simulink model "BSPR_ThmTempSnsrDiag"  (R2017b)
settings: Solver=FixedStepDiscrete  StartTime=0.0  StopTime=10.0  FixedStep=0.02  RelTol=1e-3  EnableMultiTasking=on
undefined symbols (not defined in the file): BCCR_cntClntTempDiag_CW, bin2dec, BSPR_tClntDsTOvrTemp_C, BSPR_tClntUsTOvrTemp_C, BSPR_tiClntDsTElecMax_C, BSPR_tiClntDsTElecMin_C, BSPR_tiClntDsTJit_C, BSPR_tiClntDsTOvrTemp_C, BSPR_tiClntDsTVld_C, BSPR_tiClntUsTElecMax_C, BSPR_tiClntUsTElecMin_C, BSPR_tiClntUsTJit_C, BSPR_tiClntUsTOvrTemp_C, BSPR_tiClntUsTVld_C, BSPR_uClntDsTElecMax_C, BSPR_uClntDsTElecMin_C, BSPR_uClntDsTJitDiff_C, BSPR_uClntUsTElecMax_C, BSPR_uClntUsTElecMin_C, BSPR_uClntUsTJitDiff_C
libraries: simulink x64
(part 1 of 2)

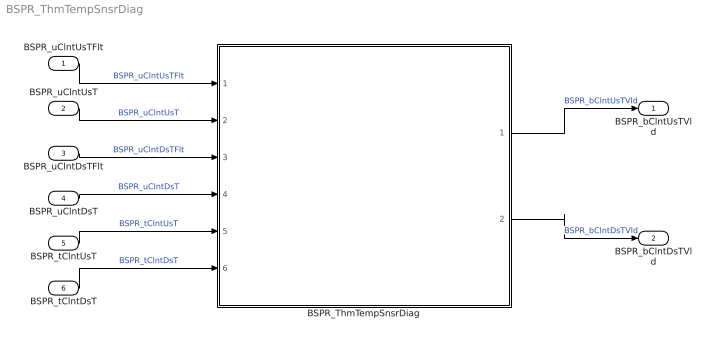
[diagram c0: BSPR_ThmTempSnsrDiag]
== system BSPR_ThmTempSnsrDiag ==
  BSPR_uClntUsTFlt : Inport
  BSPR_uClntUsT : Inport  Port=2
  BSPR_uClntDsTFlt : Inport  Port=3
  BSPR_uClntDsT : Inport  Port=4
  BSPR_tClntUsT : Inport  Port=5
  BSPR_tClntDsT : Inport  Port=6
  BSPR_ThmTempSnsrDiag : Subsystem
  BSPR_bClntUsTVld : Outport
  BSPR_bClntDsTVld : Outport  Port=2
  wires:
  BSPR_uClntUsTFlt/1 -> BSPR_ThmTempSnsrDiag/1(BSPR_uClntUsTFlt)  "BSPR_uClntUsTFlt"
  BSPR_uClntUsT/1 -> BSPR_ThmTempSnsrDiag/2(BSPR_uClntUsT)  "BSPR_uClntUsT"
  BSPR_uClntDsTFlt/1 -> BSPR_ThmTempSnsrDiag/3(BSPR_uClntDsTFlt)  "BSPR_uClntDsTFlt"
  BSPR_uClntDsT/1 -> BSPR_ThmTempSnsrDiag/4(BSPR_uClntDsT)  "BSPR_uClntDsT"
  BSPR_ThmTempSnsrDiag/1(BSPR_bClntUsTVld) -> BSPR_bClntUsTVld/1  "BSPR_bClntUsTVld"
  BSPR_ThmTempSnsrDiag/2(BSPR_bClntDsTVld) -> BSPR_bClntDsTVld/1  "BSPR_bClntDsTVld"
  BSPR_tClntUsT/1 -> BSPR_ThmTempSnsrDiag/5(BSPR_tClntUsT)  "BSPR_tClntUsT"
  BSPR_tClntDsT/1 -> BSPR_ThmTempSnsrDiag/6(BSPR_tClntDsT)  "BSPR_tClntDsT"

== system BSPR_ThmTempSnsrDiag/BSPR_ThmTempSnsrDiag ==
  BSPR_uClntUsTFlt : Inport
  BSPR_uClntUsT : Inport  Port=2
  BSPR_uClntDsTFlt : Inport  Port=3
  BSPR_uClntDsT : Inport  Port=4
  BSPR_tClntUsT : Inport  Port=5
  BSPR_tClntDsT : Inport  Port=6
  CIntDsTErrChk : Subsystem
  CIntTempDsmRpt : Subsystem
  CIntUsTErrChk : Subsystem
  BSPR_bClntUsTVld : Outport
  BSPR_bClntDsTVld : Outport  Port=2
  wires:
  BSPR_uClntUsTFlt/1 -> CIntUsTErrChk/1(BSPR_uClntUsTFlt)
  BSPR_uClntUsT/1 -> CIntUsTErrChk/2(BSPR_uClntUsT)
  CIntUsTErrChk/1(BSPR_bClntUsTJitErrStt) -> CIntTempDsmRpt/1(BSPR_bClntUsTJitErrStt)
  CIntUsTErrChk/2(BSPR_bClntUsTMaxErrStt) -> CIntTempDsmRpt/2(BSPR_bClntUsTMaxErrStt)
  CIntUsTErrChk/3(BSPR_bClntUsTMinErrStt) -> CIntTempDsmRpt/3(BSPR_bClntUsTMinErrStt)
  CIntUsTErrChk/4(BSPR_bClntUsTJitErrDet) -> CIntTempDsmRpt/4(BSPR_bClntUsTJitErrDet)
  CIntUsTErrChk/5(BSPR_bClntUsTJitErrHeal) -> CIntTempDsmRpt/5(BSPR_bClntUsTJitErrHeal)
  CIntUsTErrChk/6(BSPR_bClntUsTMaxErrDet) -> CIntTempDsmRpt/6(BSPR_bClntUsTMaxErrDet)
  CIntUsTErrChk/7(BSPR_bClntUsTMaxErrHeal) -> CIntTempDsmRpt/7(BSPR_bClntUsTMaxErrHeal)
  CIntUsTErrChk/8(BSPR_bClntUsTMinErrDet) -> CIntTempDsmRpt/8(BSPR_bClntUsTMinErrDet)
  CIntUsTErrChk/9(BSPR_bClntUsTMinErrHeal) -> CIntTempDsmRpt/9(BSPR_bClntUsTMinErrHeal)
  CIntTempDsmRpt/1(BSPR_bClntUsTVld) -> BSPR_bClntUsTVld/1
  BSPR_uClntDsTFlt/1 -> CIntDsTErrChk/2(BSPR_uClntDsTFlt)
  BSPR_uClntDsT/1 -> CIntDsTErrChk/3(BSPR_uClntDsT)
  CIntTempDsmRpt/2(BSPR_bClntDsTVld) -> BSPR_bClntDsTVld/1
  CIntDsTErrChk/1(BSPR_bClntDsTJitErrStt) -> CIntTempDsmRpt/12(BSPR_bClntDsTJitErrStt)
  CIntDsTErrChk/2(BSPR_bClntDsTMaxErrStt) -> CIntTempDsmRpt/13(BSPR_bClntDsTMaxErrStt)
  CIntDsTErrChk/3(BSPR_bClntDsTMinErrStt) -> CIntTempDsmRpt/14(BSPR_bClntDsTMinErrStt)
  CIntDsTErrChk/4(BSPR_bClntDsTJitErrDet) -> CIntTempDsmRpt/15(BSPR_bClntDsTJitErrDet)
  CIntDsTErrChk/5(BSPR_bClntDsTJitErrHeal) -> CIntTempDsmRpt/16(BSPR_bClntDsTJitErrHeal)
  CIntDsTErrChk/6(BSPR_bClntDsTMaxErrDet) -> CIntTempDsmRpt/17(BSPR_bClntDsTMaxErrDet)
  CIntDsTErrChk/7(BSPR_bClntDsTMaxErrHeal) -> CIntTempDsmRpt/18(BSPR_bClntDsTMaxErrHeal)
  CIntDsTErrChk/8(BSPR_bClntDsTMinErrDet) -> CIntTempDsmRpt/19(BSPR_bClntDsTMinErrDet)
  CIntDsTErrChk/9(BSPR_bClntDsTMinErrHeal) -> CIntTempDsmRpt/20(BSPR_bClntDsTMinErrHeal)
  BSPR_tClntUsT/1 -> CIntUsTErrChk/3(BSPR_tClntUsT)
  BSPR_tClntDsT/1 -> CIntDsTErrChk/1(BSPR_tClntDsT)
  CIntUsTErrChk/10(BSPR_bClntUsTOTErrDet) -> CIntTempDsmRpt/10(BSPR_bClntUsTOTErrDet)
  CIntUsTErrChk/11(BSPR_bClntUsTOTErrHeal) -> CIntTempDsmRpt/11(BSPR_bClntUsTOTErrHeal)
  CIntDsTErrChk/10(BSPR_bClntDsTOTErrDet) -> CIntTempDsmRpt/21(BSPR_bClntDsTOTErrDet)
  CIntDsTErrChk/11(BSPR_bClntDsTOTErrHeal) -> CIntTempDsmRpt/22(BSPR_bClntDsTOTErrHeal)

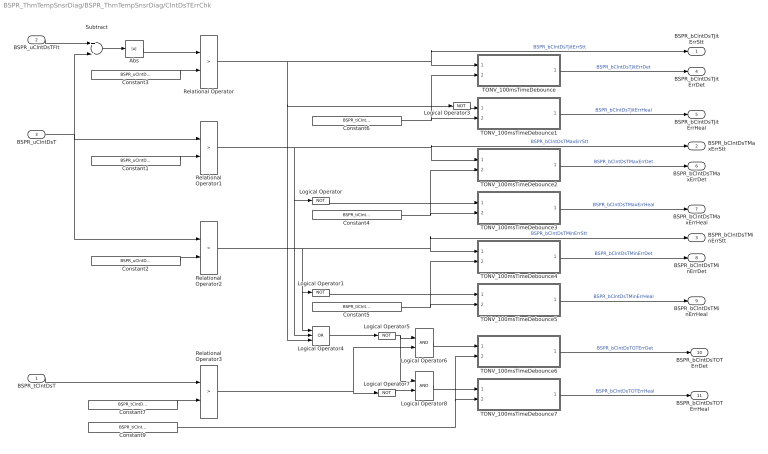
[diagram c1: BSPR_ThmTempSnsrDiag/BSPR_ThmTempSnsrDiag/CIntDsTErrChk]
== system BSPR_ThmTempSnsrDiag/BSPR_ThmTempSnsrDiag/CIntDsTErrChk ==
  BSPR_tClntDsT : Inport
  BSPR_uClntDsTFlt : Inport  Port=2
  BSPR_uClntDsT : Inport  Port=3
  Abs : Abs
  Constant1 : Constant  Value=BSPR_uClntDsTElecMax_C  OutDataTypeStr=single
  Constant2 : Constant  Value=BSPR_uClntDsTElecMin_C  OutDataTypeStr=single
  Constant3 : Constant  Value=BSPR_uClntDsTJitDiff_C  OutDataTypeStr=single
  Constant4 : Constant  Value=BSPR_tiClntDsTElecMax_C  OutDataTypeStr=single
  Constant5 : Constant  Value=BSPR_tiClntDsTElecMin_C  OutDataTypeStr=single
  Constant6 : Constant  Value=BSPR_tiClntDsTJit_C  OutDataTypeStr=single
  Constant7 : Constant  Value=BSPR_tClntDsTOvrTemp_C  OutDataTypeStr=single
  Constant9 : Constant  Value=BSPR_tiClntDsTOvrTemp_C  OutDataTypeStr=single
  Logical Operator{,1,3,5,7} (5 alike) : Logic  Operator=NOT  AllPortsSameDT=off  OutDataTypeStr=boolean
  Logical Operator4 : Logic  Operator=OR  Inputs=3  AllPortsSameDT=off  OutDataTypeStr=boolean
  Logical Operator6 : Logic  AllPortsSameDT=off  OutDataTypeStr=boolean
  Logical Operator8 : Logic  AllPortsSameDT=off  OutDataTypeStr=boolean
  Relational Operator : RelationalOperator  Operator=>  OutDataTypeStr=boolean  RndMeth=Simplest
  Relational Operator1 : RelationalOperator  Operator=>  OutDataTypeStr=boolean  RndMeth=Simplest
  Relational Operator2 : RelationalOperator  Operator=<  OutDataTypeStr=boolean  RndMeth=Simplest
  Relational Operator3 : RelationalOperator  Operator=>  OutDataTypeStr=boolean  RndMeth=Simplest
  Subtract : Sum  Inputs=+-
  TONV_100msTimeDebounce : Subsystem  TreatAsAtomicUnit=on  RTWFcnName=TONV_100msTimeDebounce  RTWFileName=SrvLib
  TONV_100msTimeDebounce1 : Subsystem  TreatAsAtomicUnit=on  RTWFcnName=TONV_100msTimeDebounce  RTWFileName=SrvLib
  TONV_100msTimeDebounce2 : Subsystem  TreatAsAtomicUnit=on  RTWFcnName=TONV_100msTimeDebounce  RTWFileName=SrvLib
  TONV_100msTimeDebounce3 : Subsystem  TreatAsAtomicUnit=on  RTWFcnName=TONV_100msTimeDebounce  RTWFileName=SrvLib
  TONV_100msTimeDebounce4 : Subsystem  TreatAsAtomicUnit=on  RTWFcnName=TONV_100msTimeDebounce  RTWFileName=SrvLib
  TONV_100msTimeDebounce5 : Subsystem  TreatAsAtomicUnit=on  RTWFcnName=TONV_100msTimeDebounce  RTWFileName=SrvLib
  TONV_100msTimeDebounce6 : Subsystem  TreatAsAtomicUnit=on  RTWFcnName=TONV_100msTimeDebounce  RTWFileName=SrvLib
  TONV_100msTimeDebounce7 : Subsystem  TreatAsAtomicUnit=on  RTWFcnName=TONV_100msTimeDebounce  RTWFileName=SrvLib
  BSPR_bClntDsTJitErrStt : Outport
  BSPR_bClntDsTMaxErrStt : Outport  Port=2
  BSPR_bClntDsTMinErrStt : Outport  Port=3
  BSPR_bClntDsTJitErrDet : Outport  Port=4
  BSPR_bClntDsTJitErrHeal : Outport  Port=5
  BSPR_bClntDsTMaxErrDet : Outport  Port=6
  BSPR_bClntDsTMaxErrHeal : Outport  Port=7
  BSPR_bClntDsTMinErrDet : Outport  Port=8
  BSPR_bClntDsTMinErrHeal : Outport  Port=9
  BSPR_bClntDsTOTErrDet : Outport  Port=10
  BSPR_bClntDsTOTErrHeal : Outport  Port=11
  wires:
  TONV_100msTimeDebounce2/1(y) -> BSPR_bClntDsTMaxErrDet/1  "BSPR_bClntDsTMaxErrDet"
  TONV_100msTimeDebounce1/1(y) -> BSPR_bClntDsTJitErrHeal/1  "BSPR_bClntDsTJitErrHeal"
  TONV_100msTimeDebounce3/1(y) -> BSPR_bClntDsTMaxErrHeal/1  "BSPR_bClntDsTMaxErrHeal"
  TONV_100msTimeDebounce4/1(y) -> BSPR_bClntDsTMinErrDet/1  "BSPR_bClntDsTMinErrDet"
  Logical Operator/1 -> TONV_100msTimeDebounce3/1(u)
  Constant4/1 -> TONV_100msTimeDebounce2/2(T), TONV_100msTimeDebounce3/2(T)
  BSPR_uClntDsT/1 -> Relational Operator2/1, Relational Operator1/1, Subtract/2
  Relational Operator1/1 -> TONV_100msTimeDebounce2/1(u), BSPR_bClntDsTMaxErrStt/1, Logical Operator4/2, Logical Operator/1  "BSPR_bClntDsTMaxErrStt"
  Constant1/1 -> Relational Operator1/2
  Constant2/1 -> Relational Operator2/2
  Constant6/1 -> TONV_100msTimeDebounce/2(T), TONV_100msTimeDebounce1/2(T)
  Relational Operator/1 -> TONV_100msTimeDebounce/1(u), BSPR_bClntDsTJitErrStt/1, Logical Operator4/3, Logical Operator3/1  "BSPR_bClntDsTJitErrStt"
  BSPR_uClntDsTFlt/1 -> Subtract/1
  Subtract/1 -> Abs/1
  Abs/1 -> Relational Operator/1
  Constant3/1 -> Relational Operator/2
  TONV_100msTimeDebounce/1(y) -> BSPR_bClntDsTJitErrDet/1  "BSPR_bClntDsTJitErrDet"
  Constant5/1 -> TONV_100msTimeDebounce4/2(T), TONV_100msTimeDebounce5/2(T)
  TONV_100msTimeDebounce5/1(y) -> BSPR_bClntDsTMinErrHeal/1  "BSPR_bClntDsTMinErrHeal"
  Logical Operator1/1 -> TONV_100msTimeDebounce5/1(u)
  Relational Operator2/1 -> Logical Operator4/1, Logical Operator1/1, BSPR_bClntDsTMinErrStt/1, TONV_100msTimeDebounce4/1(u)  "BSPR_bClntDsTMinErrStt"
  Logical Operator3/1 -> TONV_100msTimeDebounce1/1(u)
  Logical Operator4/1 -> Logical Operator5/1
  Constant7/1 -> Relational Operator3/2
  BSPR_tClntDsT/1 -> Relational Operator3/1
  Logical Operator5/1 -> Logical Operator8/1, Logical Operator6/1
  Relational Operator3/1 -> Logical Operator6/2, Logical Operator7/1
  Logical Operator6/1 -> TONV_100msTimeDebounce6/1(u)
  Logical Operator8/1 -> TONV_100msTimeDebounce7/1(u)
  Constant9/1 -> TONV_100msTimeDebounce6/2(T), TONV_100msTimeDebounce7/2(T)
  TONV_100msTimeDebounce6/1(y) -> BSPR_bClntDsTOTErrDet/1  "BSPR_bClntDsTOTErrDet"
  TONV_100msTimeDebounce7/1(y) -> BSPR_bClntDsTOTErrHeal/1  "BSPR_bClntDsTOTErrHeal"
  Logical Operator7/1 -> Logical Operator8/2

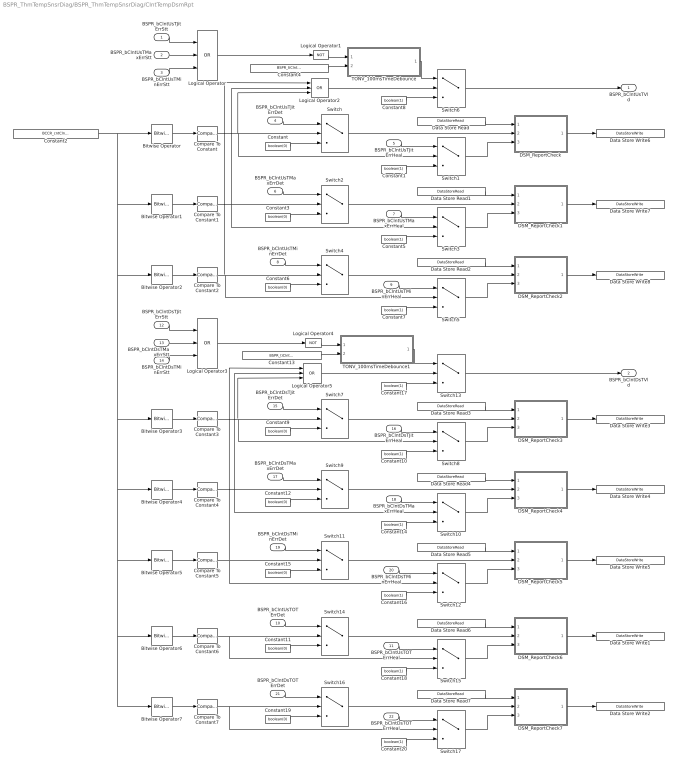
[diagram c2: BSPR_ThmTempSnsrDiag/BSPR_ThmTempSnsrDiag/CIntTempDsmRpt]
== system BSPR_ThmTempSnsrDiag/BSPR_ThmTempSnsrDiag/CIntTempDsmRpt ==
  BSPR_bClntUsTJitErrStt : Inport
  BSPR_bClntUsTMaxErrStt : Inport  Port=2
  BSPR_bClntUsTMinErrStt : Inport  Port=3
  BSPR_bClntUsTJitErrDet : Inport  Port=4
  BSPR_bClntUsTJitErrHeal : Inport  Port=5
  BSPR_bClntUsTMaxErrDet : Inport  Port=6
  BSPR_bClntUsTMaxErrHeal : Inport  Port=7
  BSPR_bClntUsTMinErrDet : Inport  Port=8
  BSPR_bClntUsTMinErrHeal : Inport  Port=9
  BSPR_bClntUsTOTErrDet : Inport  Port=10
  BSPR_bClntUsTOTErrHeal : Inport  Port=11
  BSPR_bClntDsTJitErrStt : Inport  Port=12
  BSPR_bClntDsTMaxErrStt : Inport  Port=13
  BSPR_bClntDsTMinErrStt : Inport  Port=14
  BSPR_bClntDsTJitErrDet : Inport  Port=15
  BSPR_bClntDsTJitErrHeal : Inport  Port=16
  BSPR_bClntDsTMaxErrDet : Inport  Port=17
  BSPR_bClntDsTMaxErrHeal : Inport  Port=18
  BSPR_bClntDsTMinErrDet : Inport  Port=19
  BSPR_bClntDsTMinErrHeal : Inport  Port=20
  BSPR_bClntDsTOTErrDet : Inport  Port=21
  BSPR_bClntDsTOTErrHeal : Inport  Port=22
  Bitwise Operator : simulink/Logic and Bit Operations/Bitwise Operator  logicop=AND  UseBitMask=on  BitMask=bin2dec('00000001')  BitMaskRealWorld=Stored Integer
  Bitwise Operator1 : simulink/Logic and Bit Operations/Bitwise Operator  logicop=AND  UseBitMask=on  BitMask=bin2dec('00000010')  BitMaskRealWorld=Stored Integer
  Bitwise Operator2 : simulink/Logic and Bit Operations/Bitwise Operator  logicop=AND  UseBitMask=on  BitMask=bin2dec('00000100')  BitMaskRealWorld=Stored Integer
  Bitwise Operator3 : simulink/Logic and Bit Operations/Bitwise Operator  logicop=AND  UseBitMask=on  BitMask=bin2dec('00001000')  BitMaskRealWorld=Stored Integer
  Bitwise Operator4 : simulink/Logic and Bit Operations/Bitwise Operator  logicop=AND  UseBitMask=on  BitMask=bin2dec('00010000')  BitMaskRealWorld=Stored Integer
  Bitwise Operator5 : simulink/Logic and Bit Operations/Bitwise Operator  logicop=AND  UseBitMask=on  BitMask=bin2dec('00100000')  BitMaskRealWorld=Stored Integer
  Bitwise Operator6 : simulink/Logic and Bit Operations/Bitwise Operator  logicop=AND  UseBitMask=on  BitMask=bin2dec('01000000')  BitMaskRealWorld=Stored Integer
  Bitwise Operator7 : simulink/Logic and Bit Operations/Bitwise Operator  logicop=AND  UseBitMask=on  BitMask=bin2dec('10000000')  BitMaskRealWorld=Stored Integer
  Compare To Constant : simulink/Logic and Bit Operations/Compare To Constant  relop===  const=1  OutDataTypeStr=boolean
  Compare To Constant1 : simulink/Logic and Bit Operations/Compare To Constant  relop===  const=2  OutDataTypeStr=boolean
  Compare To Constant2 : simulink/Logic and Bit Operations/Compare To Constant  relop===  const=4  OutDataTypeStr=boolean
  Compare To Constant3 : simulink/Logic and Bit Operations/Compare To Constant  relop===  const=8  OutDataTypeStr=boolean
  Compare To Constant4 : simulink/Logic and Bit Operations/Compare To Constant  relop===  const=16  OutDataTypeStr=boolean
  Compare To Constant5 : simulink/Logic and Bit Operations/Compare To Constant  relop===  const=32  OutDataTypeStr=boolean
  Compare To Constant6 : simulink/Logic and Bit Operations/Compare To Constant  relop===  const=64  OutDataTypeStr=boolean
  Compare To Constant7 : simulink/Logic and Bit Operations/Compare To Constant  relop===  const=128  OutDataTypeStr=boolean
  Constant{,3,6,9,11..12,15,19} (8 alike) : Constant  Value=boolean(0)  OutDataTypeStr=boolean
  Constant{1,5,7..8,10,14,16..18,20} (10 alike) : Constant  Value=boolean(1)  OutDataTypeStr=boolean
  Constant13 : Constant  Value=BSPR_tiClntDsTVld_C  OutDataTypeStr=single
  Constant2 : Constant  Value=BCCR_cntClntTempDiag_CW
  Constant4 : Constant  Value=BSPR_tiClntUsTVld_C  OutDataTypeStr=single
  DSM_ReportCheck : Subsystem  TreatAsAtomicUnit=on  RTWFcnName=DSM_ReportCheck  RTWFileName=SrvLib
  DSM_ReportCheck1 : Subsystem  TreatAsAtomicUnit=on  RTWFcnName=DSM_ReportCheck  RTWFileName=SrvLib
  DSM_ReportCheck2 : Subsystem  TreatAsAtomicUnit=on  RTWFcnName=DSM_ReportCheck  RTWFileName=SrvLib
  DSM_ReportCheck3 : Subsystem  TreatAsAtomicUnit=on  RTWFcnName=DSM_ReportCheck  RTWFileName=SrvLib
  DSM_ReportCheck4 : Subsystem  TreatAsAtomicUnit=on  RTWFcnName=DSM_ReportCheck  RTWFileName=SrvLib
  DSM_ReportCheck5 : Subsystem  TreatAsAtomicUnit=on  RTWFcnName=DSM_ReportCheck  RTWFileName=SrvLib
  DSM_ReportCheck6 : Subsystem  TreatAsAtomicUnit=on  RTWFcnName=DSM_ReportCheck  RTWFileName=SrvLib
  DSM_ReportCheck7 : Subsystem  TreatAsAtomicUnit=on  RTWFcnName=DSM_ReportCheck  RTWFileName=SrvLib
  Data Store Read : DataStoreRead  DataStoreName=DFC_ClntUsTElecSig
  Data Store Read1 : DataStoreRead  DataStoreName=DFC_ClntUsTElecMax
  Data Store Read2 : DataStoreRead  DataStoreName=DFC_ClntUsTElecMin
  Data Store Read3 : DataStoreRead  DataStoreName=DFC_ClntDsTElecSig
  Data Store Read4 : DataStoreRead  DataStoreName=DFC_ClntDsTElecMax
  Data Store Read5 : DataStoreRead  DataStoreName=DFC_ClntDsTElecMin
  Data Store Read6 : DataStoreRead  DataStoreName=DFC_InClntOverTmp
  Data Store Read7 : DataStoreRead  DataStoreName=DFC_OutClntOverTmp
  Data Store Write1 : DataStoreWrite  DataStoreName=DFC_InClntOverTmp
  Data Store Write2 : DataStoreWrite  DataStoreName=DFC_OutClntOverTmp
  Data Store Write3 : DataStoreWrite  DataStoreName=DFC_ClntDsTElecSig
  Data Store Write4 : DataStoreWrite  DataStoreName=DFC_ClntDsTElecMax
  Data Store Write5 : DataStoreWrite  DataStoreName=DFC_ClntDsTElecMin
  Data Store Write6 : DataStoreWrite  DataStoreName=DFC_ClntUsTElecSig
  Data Store Write7 : DataStoreWrite  DataStoreName=DFC_ClntUsTElecMax
  Data Store Write8 : DataStoreWrite  DataStoreName=DFC_ClntUsTElecMin
  Logical Operator{,2..3,5} (4 alike) : Logic  Operator=OR  Inputs=3  AllPortsSameDT=off  OutDataTypeStr=boolean
  Logical Operator1 : Logic  Operator=NOT  AllPortsSameDT=off  OutDataTypeStr=boolean
  Logical Operator4 : Logic  Operator=NOT  AllPortsSameDT=off  OutDataTypeStr=boolean
  Switch{,1..17} (18 alike) : Switch  Criteria=u2 > Threshold
  TONV_100msTimeDebounce : Subsystem  TreatAsAtomicUnit=on  RTWFcnName=TONV_100msTimeDebounce  RTWFileName=SrvLib
  TONV_100msTimeDebounce1 : Subsystem  TreatAsAtomicUnit=on  RTWFcnName=TONV_100msTimeDebounce  RTWFileName=SrvLib
  BSPR_bClntUsTVld : Outport
  BSPR_bClntDsTVld : Outport  Port=2
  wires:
  BSPR_bClntUsTJitErrStt/1 -> Logical Operator/1
  BSPR_bClntUsTMaxErrStt/1 -> Logical Operator/2
  BSPR_bClntUsTMinErrStt/1 -> Logical Operator/3
  Logical Operator/1 -> Logical Operator1/1
  Logical Operator1/1 -> TONV_100msTimeDebounce/1(u)
  Switch6/1 -> BSPR_bClntUsTVld/1
  Constant4/1 -> TONV_100msTimeDebounce/2(T)
  Constant/1 -> Switch/3
  BSPR_bClntUsTJitErrDet/1 -> Switch/1
  BSPR_bClntUsTJitErrHeal/1 -> Switch1/1
  Constant1/1 -> Switch1/3
  Switch1/1 -> DSM_ReportCheck/3(Heal)
  Switch/1 -> DSM_ReportCheck/2(Err)
  Bitwise Operator/1 -> Compare To Constant/1
  Compare To Constant/1 -> Logical Operator2/3, Switch1/2, Switch/2
  Constant3/1 -> Switch2/3
  Constant5/1 -> Switch3/3
  Switch3/1 -> DSM_ReportCheck1/3(Heal)
  Switch2/1 -> DSM_ReportCheck1/2(Err)
  BSPR_bClntUsTMaxErrHeal/1 -> Switch3/1
  BSPR_bClntUsTMaxErrDet/1 -> Switch2/1
  Bitwise Operator1/1 -> Compare To Constant1/1
  Compare To Constant1/1 -> Switch2/2, Switch3/2, Logical Operator2/2
  Data Store Read1/1 -> DSM_ReportCheck1/1(Dfc_id_nv)
  Data Store Read/1 -> DSM_ReportCheck/1(Dfc_id_nv)
  Constant6/1 -> Switch4/3
  Constant7/1 -> Switch5/3
  Switch5/1 -> DSM_ReportCheck2/3(Heal)
  Switch4/1 -> DSM_ReportCheck2/2(Err)
  BSPR_bClntUsTMinErrHeal/1 -> Switch5/1
  BSPR_bClntUsTMinErrDet/1 -> Switch4/1
  Bitwise Operator2/1 -> Compare To Constant2/1
  Compare To Constant2/1 -> Switch4/2, Switch5/2, Logical Operator2/1
  Data Store Read2/1 -> DSM_ReportCheck2/1(Dfc_id_nv)
  DSM_ReportCheck/1(Dfc_id) -> Data Store Write6/1
  DSM_ReportCheck1/1(Dfc_id) -> Data Store Write7/1
  DSM_ReportCheck2/1(Dfc_id) -> Data Store Write8/1
  TONV_100msTimeDebounce/1(y) -> Switch6/1
  Constant8/1 -> Switch6/3
  Logical Operator2/1 -> Switch6/2
  Logical Operator5/1 -> Switch13/2
  Constant17/1 -> Switch13/3
  TONV_100msTimeDebounce1/1(y) -> Switch13/1
  DSM_ReportCheck5/1(Dfc_id) -> Data Store Write5/1
  DSM_ReportCheck4/1(Dfc_id) -> Data Store Write4/1
  DSM_ReportCheck3/1(Dfc_id) -> Data Store Write3/1
  Data Store Read5/1 -> DSM_ReportCheck5/1(Dfc_id_nv)
  Compare To Constant5/1 -> Switch11/2, Switch12/2, Logical Operator5/1
  Bitwise Operator5/1 -> Compare To Constant5/1
  BSPR_bClntDsTMinErrDet/1 -> Switch11/1
  BSPR_bClntDsTMinErrHeal/1 -> Switch12/1
  Switch11/1 -> DSM_ReportCheck5/2(Err)
  Switch12/1 -> DSM_ReportCheck5/3(Heal)
  Constant16/1 -> Switch12/3
  Constant15/1 -> Switch11/3
  Data Store Read3/1 -> DSM_ReportCheck3/1(Dfc_id_nv)
  Data Store Read4/1 -> DSM_ReportCheck4/1(Dfc_id_nv)
  Compare To Constant4/1 -> Switch9/2, Switch10/2, Logical Operator5/2
  Bitwise Operator4/1 -> Compare To Constant4/1
  BSPR_bClntDsTMaxErrDet/1 -> Switch9/1
  BSPR_bClntDsTMaxErrHeal/1 -> Switch10/1
  Switch9/1 -> DSM_ReportCheck4/2(Err)
  Switch10/1 -> DSM_ReportCheck4/3(Heal)
  Constant14/1 -> Switch10/3
  Constant12/1 -> Switch9/3
  Compare To Constant3/1 -> Logical Operator5/3, Switch7/2, Switch8/2
  Bitwise Operator3/1 -> Compare To Constant3/1
  Switch7/1 -> DSM_ReportCheck3/2(Err)
  Switch8/1 -> DSM_ReportCheck3/3(Heal)
  Constant10/1 -> Switch8/3
  BSPR_bClntDsTJitErrHeal/1 -> Switch8/1
  BSPR_bClntDsTJitErrDet/1 -> Switch7/1
  Constant9/1 -> Switch7/3
  Constant13/1 -> TONV_100msTimeDebounce1/2(T)
  Switch13/1 -> BSPR_bClntDsTVld/1
  Logical Operator4/1 -> TONV_100msTimeDebounce1/1(u)
  Logical Operator3/1 -> Logical Operator4/1
  BSPR_bClntDsTMinErrStt/1 -> Logical Operator3/3
  BSPR_bClntDsTMaxErrStt/1 -> Logical Operator3/2
  BSPR_bClntDsTJitErrStt/1 -> Logical Operator3/1
  Constant2/1 -> Bitwise Operator/1, Bitwise Operator1/1, Bitwise Operator2/1, Bitwise Operator3/1, Bitwise Operator4/1, Bitwise Operator7/1, Bitwise Operator6/1, Bitwise Operator5/1
  DSM_ReportCheck6/1(Dfc_id) -> Data Store Write1/1
  Data Store Read6/1 -> DSM_ReportCheck6/1(Dfc_id_nv)
  Compare To Constant6/1 -> Switch15/2, Switch14/2
  Bitwise Operator6/1 -> Compare To Constant6/1
  BSPR_bClntUsTOTErrDet/1 -> Switch14/1
  BSPR_bClntUsTOTErrHeal/1 -> Switch15/1
  Switch14/1 -> DSM_ReportCheck6/2(Err)
  Switch15/1 -> DSM_ReportCheck6/3(Heal)
  Constant18/1 -> Switch15/3
  Constant11/1 -> Switch14/3
  DSM_ReportCheck7/1(Dfc_id) -> Data Store Write2/1
  Data Store Read7/1 -> DSM_ReportCheck7/1(Dfc_id_nv)
  Compare To Constant7/1 -> Switch16/2, Switch17/2
  Bitwise Operator7/1 -> Compare To Constant7/1
  BSPR_bClntDsTOTErrDet/1 -> Switch16/1
  BSPR_bClntDsTOTErrHeal/1 -> Switch17/1
  Switch16/1 -> DSM_ReportCheck7/2(Err)
  Switch17/1 -> DSM_ReportCheck7/3(Heal)
  Constant20/1 -> Switch17/3
  Constant19/1 -> Switch16/3

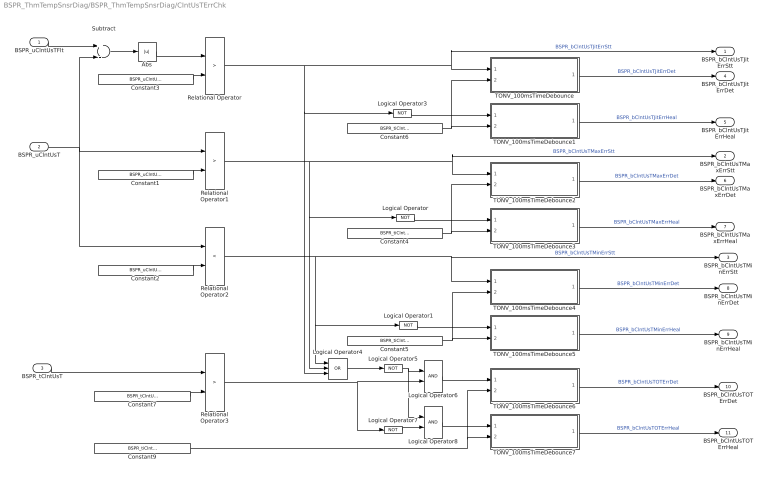
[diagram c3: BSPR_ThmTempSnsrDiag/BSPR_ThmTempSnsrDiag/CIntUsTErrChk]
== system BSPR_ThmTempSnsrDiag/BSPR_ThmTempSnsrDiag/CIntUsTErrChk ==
  BSPR_uClntUsTFlt : Inport
  BSPR_uClntUsT : Inport  Port=2
  BSPR_tClntUsT : Inport  Port=3
  Abs : Abs
  Constant1 : Constant  Value=BSPR_uClntUsTElecMax_C  OutDataTypeStr=single
  Constant2 : Constant  Value=BSPR_uClntUsTElecMin_C  OutDataTypeStr=single
  Constant3 : Constant  Value=BSPR_uClntUsTJitDiff_C  OutDataTypeStr=single
  Constant4 : Constant  Value=BSPR_tiClntUsTElecMax_C  OutDataTypeStr=single
  Constant5 : Constant  Value=BSPR_tiClntUsTElecMin_C  OutDataTypeStr=single
  Constant6 : Constant  Value=BSPR_tiClntUsTJit_C  OutDataTypeStr=single
  Constant7 : Constant  Value=BSPR_tClntUsTOvrTemp_C  OutDataTypeStr=single
  Constant9 : Constant  Value=BSPR_tiClntUsTOvrTemp_C  OutDataTypeStr=single
  Logical Operator{,1,3,5,7} (5 alike) : Logic  Operator=NOT  AllPortsSameDT=off  OutDataTypeStr=boolean
  Logical Operator4 : Logic  Operator=OR  Inputs=3  AllPortsSameDT=off  OutDataTypeStr=boolean
  Logical Operator6 : Logic  AllPortsSameDT=off  OutDataTypeStr=boolean
  Logical Operator8 : Logic  AllPortsSameDT=off  OutDataTypeStr=boolean
  Relational Operator : RelationalOperator  Operator=>  OutDataTypeStr=boolean  RndMeth=Simplest
  Relational Operator1 : RelationalOperator  Operator=>  OutDataTypeStr=boolean  RndMeth=Simplest
  Relational Operator2 : RelationalOperator  Operator=<  OutDataTypeStr=boolean  RndMeth=Simplest
  Relational Operator3 : RelationalOperator  Operator=>  OutDataTypeStr=boolean  RndMeth=Simplest
  Subtract : Sum  Inputs=+-
  TONV_100msTimeDebounce : Subsystem  TreatAsAtomicUnit=on  RTWFcnName=TONV_100msTimeDebounce  RTWFileName=SrvLib
  TONV_100msTimeDebounce1 : Subsystem  TreatAsAtomicUnit=on  RTWFcnName=TONV_100msTimeDebounce  RTWFileName=SrvLib
  TONV_100msTimeDebounce2 : Subsystem  TreatAsAtomicUnit=on  RTWFcnName=TONV_100msTimeDebounce  RTWFileName=SrvLib
  TONV_100msTimeDebounce3 : Subsystem  TreatAsAtomicUnit=on  RTWFcnName=TONV_100msTimeDebounce  RTWFileName=SrvLib
  TONV_100msTimeDebounce4 : Subsystem  TreatAsAtomicUnit=on  RTWFcnName=TONV_100msTimeDebounce  RTWFileName=SrvLib
  TONV_100msTimeDebounce5 : Subsystem  TreatAsAtomicUnit=on  RTWFcnName=TONV_100msTimeDebounce  RTWFileName=SrvLib
  TONV_100msTimeDebounce6 : Subsystem  TreatAsAtomicUnit=on  RTWFcnName=TONV_100msTimeDebounce  RTWFileName=SrvLib
  TONV_100msTimeDebounce7 : Subsystem  TreatAsAtomicUnit=on  RTWFcnName=TONV_100msTimeDebounce  RTWFileName=SrvLib
  BSPR_bClntUsTJitErrStt : Outport
  BSPR_bClntUsTMaxErrStt : Outport  Port=2
  BSPR_bClntUsTMinErrStt : Outport  Port=3
  BSPR_bClntUsTJitErrDet : Outport  Port=4
  BSPR_bClntUsTJitErrHeal : Outport  Port=5
  BSPR_bClntUsTMaxErrDet : Outport  Port=6
  BSPR_bClntUsTMaxErrHeal : Outport  Port=7
  BSPR_bClntUsTMinErrDet : Outport  Port=8
  BSPR_bClntUsTMinErrHeal : Outport  Port=9
  BSPR_bClntUsTOTErrDet : Outport  Port=10
  BSPR_bClntUsTOTErrHeal : Outport  Port=11
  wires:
  Logical Operator1/1 -> TONV_100msTimeDebounce5/1(u)
  TONV_100msTimeDebounce5/1(y) -> BSPR_bClntUsTMinErrHeal/1  "BSPR_bClntUsTMinErrHeal"
  Constant5/1 -> TONV_100msTimeDebounce5/2(T), TONV_100msTimeDebounce4/2(T)
  TONV_100msTimeDebounce/1(y) -> BSPR_bClntUsTJitErrDet/1  "BSPR_bClntUsTJitErrDet"
  Constant3/1 -> Relational Operator/2
  Abs/1 -> Relational Operator/1
  Subtract/1 -> Abs/1
  BSPR_uClntUsTFlt/1 -> Subtract/1
  Relational Operator/1 -> BSPR_bClntUsTJitErrStt/1, TONV_100msTimeDebounce/1(u), Logical Operator4/3, Logical Operator3/1  "BSPR_bClntUsTJitErrStt"
  Constant6/1 -> TONV_100msTimeDebounce/2(T), TONV_100msTimeDebounce1/2(T)
  Constant2/1 -> Relational Operator2/2
  Constant1/1 -> Relational Operator1/2
  Relational Operator1/1 -> TONV_100msTimeDebounce2/1(u), BSPR_bClntUsTMaxErrStt/1, Logical Operator4/2, Logical Operator/1  "BSPR_bClntUsTMaxErrStt"
  BSPR_uClntUsT/1 -> Subtract/2, Relational Operator2/1, Relational Operator1/1
  Constant4/1 -> TONV_100msTimeDebounce2/2(T), TONV_100msTimeDebounce3/2(T)
  Logical Operator/1 -> TONV_100msTimeDebounce3/1(u)
  TONV_100msTimeDebounce4/1(y) -> BSPR_bClntUsTMinErrDet/1  "BSPR_bClntUsTMinErrDet"
  TONV_100msTimeDebounce3/1(y) -> BSPR_bClntUsTMaxErrHeal/1  "BSPR_bClntUsTMaxErrHeal"
  TONV_100msTimeDebounce1/1(y) -> BSPR_bClntUsTJitErrHeal/1  "BSPR_bClntUsTJitErrHeal"
  TONV_100msTimeDebounce2/1(y) -> BSPR_bClntUsTMaxErrDet/1  "BSPR_bClntUsTMaxErrDet"
  Relational Operator2/1 -> BSPR_bClntUsTMinErrStt/1, TONV_100msTimeDebounce4/1(u), Logical Operator4/1, Logical Operator1/1  "BSPR_bClntUsTMinErrStt"
  Logical Operator3/1 -> TONV_100msTimeDebounce1/1(u)
  Logical Operator4/1 -> Logical Operator5/1
  Constant7/1 -> Relational Operator3/2
  BSPR_tClntUsT/1 -> Relational Operator3/1
  Logical Operator5/1 -> Logical Operator8/1, Logical Operator6/1
  Relational Operator3/1 -> Logical Operator7/1, Logical Operator6/2
  Logical Operator6/1 -> TONV_100msTimeDebounce6/1(u)
  Logical Operator8/1 -> TONV_100msTimeDebounce7/1(u)
  Constant9/1 -> TONV_100msTimeDebounce6/2(T), TONV_100msTimeDebounce7/2(T)
  TONV_100msTimeDebounce6/1(y) -> BSPR_bClntUsTOTErrDet/1  "BSPR_bClntUsTOTErrDet"
  TONV_100msTimeDebounce7/1(y) -> BSPR_bClntUsTOTErrHeal/1  "BSPR_bClntUsTOTErrHeal"
  Logical Operator7/1 -> Logical Operator8/2

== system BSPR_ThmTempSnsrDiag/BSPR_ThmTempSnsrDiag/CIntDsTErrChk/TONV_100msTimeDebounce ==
  note: Turn On Delay Time Deboune
  u : Inport
  T : Inport  Port=2
  Add : Sum
  Constant1 : Constant  Value=0  OutDataTypeStr=single
  Constant2 : Constant  OutDataTypeStr=uint8
  Constant3 : Constant  Value=0  OutDataTypeStr=uint8
  Constant4 : Constant  Value=0.1  OutDataTypeStr=single
  Delay : Delay  DelayLength=1  InitialCondition=0
  MinMax : MinMax  Inputs=2
  Product : Product  OutMin=[0]  OutMax=[65535]  OutDataTypeStr=single
  Relational Operator : RelationalOperator  Operator=>  OutDataTypeStr=boolean  RndMeth=Simplest
  Switch : Switch  Criteria=u2 ~= 0
  Switch1 : Switch  Criteria=u2 ~= 0
  y : Outport
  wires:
  MinMax/1 -> Add/2
  T/1 -> Relational Operator/2, MinMax/1
  Relational Operator/1 -> y/1
  Delay/1 -> MinMax/2
  Switch/1 -> Add/1
  Product/1 -> Delay/1, Relational Operator/1
  Add/1 -> Product/2
  Constant1/1 -> Switch/3
  Constant4/1 -> Switch/1
  u/1 -> Switch/2, Switch1/2
  Constant2/1 -> Switch1/1
  Constant3/1 -> Switch1/3
  Switch1/1 -> Product/1

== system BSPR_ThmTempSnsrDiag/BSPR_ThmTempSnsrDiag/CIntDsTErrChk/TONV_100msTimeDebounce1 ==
  note: Turn On Delay Time Deboune
  u : Inport
  T : Inport  Port=2
  Add : Sum
  Constant1 : Constant  Value=0  OutDataTypeStr=single
  Constant2 : Constant  OutDataTypeStr=uint8
  Constant3 : Constant  Value=0  OutDataTypeStr=uint8
  Constant4 : Constant  Value=0.1  OutDataTypeStr=single
  Delay : Delay  DelayLength=1  InitialCondition=0
  MinMax : MinMax  Inputs=2
  Product : Product  OutMin=[0]  OutMax=[65535]  OutDataTypeStr=single
  Relational Operator : RelationalOperator  Operator=>  OutDataTypeStr=boolean  RndMeth=Simplest
  Switch : Switch  Criteria=u2 ~= 0
  Switch1 : Switch  Criteria=u2 ~= 0
  y : Outport
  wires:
  Switch1/1 -> Product/1
  Constant3/1 -> Switch1/3
  Constant2/1 -> Switch1/1
  u/1 -> Switch1/2, Switch/2
  Constant4/1 -> Switch/1
  Constant1/1 -> Switch/3
  Add/1 -> Product/2
  Product/1 -> Relational Operator/1, Delay/1
  Switch/1 -> Add/1
  Delay/1 -> MinMax/2
  Relational Operator/1 -> y/1
  T/1 -> MinMax/1, Relational Operator/2
  MinMax/1 -> Add/2

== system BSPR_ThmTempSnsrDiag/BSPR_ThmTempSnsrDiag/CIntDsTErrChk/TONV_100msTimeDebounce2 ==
  note: Turn On Delay Time Deboune
  u : Inport
  T : Inport  Port=2
  Add : Sum
  Constant1 : Constant  Value=0  OutDataTypeStr=single
  Constant2 : Constant  OutDataTypeStr=uint8
  Constant3 : Constant  Value=0  OutDataTypeStr=uint8
  Constant4 : Constant  Value=0.1  OutDataTypeStr=single
  Delay : Delay  DelayLength=1  InitialCondition=0
  MinMax : MinMax  Inputs=2
  Product : Product  OutMin=[0]  OutMax=[65535]  OutDataTypeStr=single
  Relational Operator : RelationalOperator  Operator=>  OutDataTypeStr=boolean  RndMeth=Simplest
  Switch : Switch  Criteria=u2 ~= 0
  Switch1 : Switch  Criteria=u2 ~= 0
  y : Outport
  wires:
  Switch1/1 -> Product/1
  Constant3/1 -> Switch1/3
  Constant2/1 -> Switch1/1
  u/1 -> Switch1/2, Switch/2
  Constant4/1 -> Switch/1
  Constant1/1 -> Switch/3
  Add/1 -> Product/2
  Product/1 -> Relational Operator/1, Delay/1
  Switch/1 -> Add/1
  Delay/1 -> MinMax/2
  Relational Operator/1 -> y/1
  T/1 -> MinMax/1, Relational Operator/2
  MinMax/1 -> Add/2

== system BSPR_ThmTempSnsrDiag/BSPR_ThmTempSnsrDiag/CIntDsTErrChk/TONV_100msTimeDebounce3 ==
  note: Turn On Delay Time Deboune
  u : Inport
  T : Inport  Port=2
  Add : Sum
  Constant1 : Constant  Value=0  OutDataTypeStr=single
  Constant2 : Constant  OutDataTypeStr=uint8
  Constant3 : Constant  Value=0  OutDataTypeStr=uint8
  Constant4 : Constant  Value=0.1  OutDataTypeStr=single
  Delay : Delay  DelayLength=1  InitialCondition=0
  MinMax : MinMax  Inputs=2
  Product : Product  OutMin=[0]  OutMax=[65535]  OutDataTypeStr=single
  Relational Operator : RelationalOperator  Operator=>  OutDataTypeStr=boolean  RndMeth=Simplest
  Switch : Switch  Criteria=u2 ~= 0
  Switch1 : Switch  Criteria=u2 ~= 0
  y : Outport
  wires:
  MinMax/1 -> Add/2
  T/1 -> Relational Operator/2, MinMax/1
  Relational Operator/1 -> y/1
  Delay/1 -> MinMax/2
  Switch/1 -> Add/1
  Product/1 -> Delay/1, Relational Operator/1
  Add/1 -> Product/2
  Constant1/1 -> Switch/3
  Constant4/1 -> Switch/1
  u/1 -> Switch/2, Switch1/2
  Constant2/1 -> Switch1/1
  Constant3/1 -> Switch1/3
  Switch1/1 -> Product/1

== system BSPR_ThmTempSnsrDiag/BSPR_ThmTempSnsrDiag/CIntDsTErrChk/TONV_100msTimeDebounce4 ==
  note: Turn On Delay Time Deboune
  u : Inport
  T : Inport  Port=2
  Add : Sum
  Constant1 : Constant  Value=0  OutDataTypeStr=single
  Constant2 : Constant  OutDataTypeStr=uint8
  Constant3 : Constant  Value=0  OutDataTypeStr=uint8
  Constant4 : Constant  Value=0.1  OutDataTypeStr=single
  Delay : Delay  DelayLength=1  InitialCondition=0
  MinMax : MinMax  Inputs=2
  Product : Product  OutMin=[0]  OutMax=[65535]  OutDataTypeStr=single
  Relational Operator : RelationalOperator  Operator=>  OutDataTypeStr=boolean  RndMeth=Simplest
  Switch : Switch  Criteria=u2 ~= 0
  Switch1 : Switch  Criteria=u2 ~= 0
  y : Outport
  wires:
  MinMax/1 -> Add/2
  T/1 -> Relational Operator/2, MinMax/1
  Relational Operator/1 -> y/1
  Delay/1 -> MinMax/2
  Switch/1 -> Add/1
  Product/1 -> Delay/1, Relational Operator/1
  Add/1 -> Product/2
  Constant1/1 -> Switch/3
  Constant4/1 -> Switch/1
  u/1 -> Switch/2, Switch1/2
  Constant2/1 -> Switch1/1
  Constant3/1 -> Switch1/3
  Switch1/1 -> Product/1

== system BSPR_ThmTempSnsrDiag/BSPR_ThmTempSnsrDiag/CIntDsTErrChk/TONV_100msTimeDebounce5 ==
  note: Turn On Delay Time Deboune
  u : Inport
  T : Inport  Port=2
  Add : Sum
  Constant1 : Constant  Value=0  OutDataTypeStr=single
  Constant2 : Constant  OutDataTypeStr=uint8
  Constant3 : Constant  Value=0  OutDataTypeStr=uint8
  Constant4 : Constant  Value=0.1  OutDataTypeStr=single
  Delay : Delay  DelayLength=1  InitialCondition=0
  MinMax : MinMax  Inputs=2
  Product : Product  OutMin=[0]  OutMax=[65535]  OutDataTypeStr=single
  Relational Operator : RelationalOperator  Operator=>  OutDataTypeStr=boolean  RndMeth=Simplest
  Switch : Switch  Criteria=u2 ~= 0
  Switch1 : Switch  Criteria=u2 ~= 0
  y : Outport
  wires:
  Switch1/1 -> Product/1
  Constant3/1 -> Switch1/3
  Constant2/1 -> Switch1/1
  u/1 -> Switch1/2, Switch/2
  Constant4/1 -> Switch/1
  Constant1/1 -> Switch/3
  Add/1 -> Product/2
  Product/1 -> Relational Operator/1, Delay/1
  Switch/1 -> Add/1
  Delay/1 -> MinMax/2
  Relational Operator/1 -> y/1
  T/1 -> MinMax/1, Relational Operator/2
  MinMax/1 -> Add/2

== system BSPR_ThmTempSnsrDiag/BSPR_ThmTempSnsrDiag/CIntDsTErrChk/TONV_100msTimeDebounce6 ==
  note: Turn On Delay Time Deboune
  u : Inport
  T : Inport  Port=2
  Add : Sum
  Constant1 : Constant  Value=0  OutDataTypeStr=single
  Constant2 : Constant  OutDataTypeStr=uint8
  Constant3 : Constant  Value=0  OutDataTypeStr=uint8
  Constant4 : Constant  Value=0.1  OutDataTypeStr=single
  Delay : Delay  DelayLength=1  InitialCondition=0
  MinMax : MinMax  Inputs=2
  Product : Product  OutMin=[0]  OutMax=[65535]  OutDataTypeStr=single
  Relational Operator : RelationalOperator  Operator=>  OutDataTypeStr=boolean  RndMeth=Simplest
  Switch : Switch  Criteria=u2 ~= 0
  Switch1 : Switch  Criteria=u2 ~= 0
  y : Outport
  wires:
  MinMax/1 -> Add/2
  T/1 -> Relational Operator/2, MinMax/1
  Relational Operator/1 -> y/1
  Delay/1 -> MinMax/2
  Switch/1 -> Add/1
  Product/1 -> Delay/1, Relational Operator/1
  Add/1 -> Product/2
  Constant1/1 -> Switch/3
  Constant4/1 -> Switch/1
  u/1 -> Switch/2, Switch1/2
  Constant2/1 -> Switch1/1
  Constant3/1 -> Switch1/3
  Switch1/1 -> Product/1

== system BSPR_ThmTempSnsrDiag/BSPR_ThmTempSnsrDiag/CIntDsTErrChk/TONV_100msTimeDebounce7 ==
  note: Turn On Delay Time Deboune
  u : Inport
  T : Inport  Port=2
  Add : Sum
  Constant1 : Constant  Value=0  OutDataTypeStr=single
  Constant2 : Constant  OutDataTypeStr=uint8
  Constant3 : Constant  Value=0  OutDataTypeStr=uint8
  Constant4 : Constant  Value=0.1  OutDataTypeStr=single
  Delay : Delay  DelayLength=1  InitialCondition=0
  MinMax : MinMax  Inputs=2
  Product : Product  OutMin=[0]  OutMax=[65535]  OutDataTypeStr=single
  Relational Operator : RelationalOperator  Operator=>  OutDataTypeStr=boolean  RndMeth=Simplest
  Switch : Switch  Criteria=u2 ~= 0
  Switch1 : Switch  Criteria=u2 ~= 0
  y : Outport
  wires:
  Switch1/1 -> Product/1
  Constant3/1 -> Switch1/3
  Constant2/1 -> Switch1/1
  u/1 -> Switch1/2, Switch/2
  Constant4/1 -> Switch/1
  Constant1/1 -> Switch/3
  Add/1 -> Product/2
  Product/1 -> Relational Operator/1, Delay/1
  Switch/1 -> Add/1
  Delay/1 -> MinMax/2
  Relational Operator/1 -> y/1
  T/1 -> MinMax/1, Relational Operator/2
  MinMax/1 -> Add/2

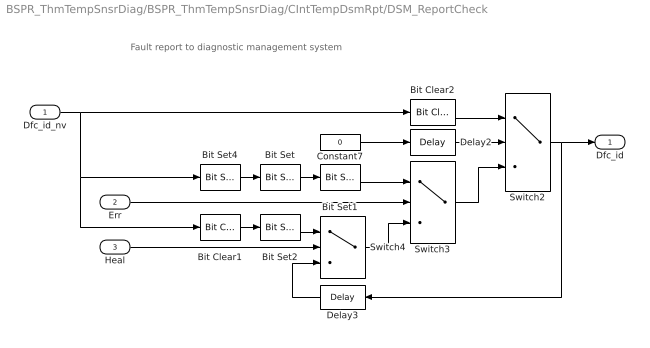
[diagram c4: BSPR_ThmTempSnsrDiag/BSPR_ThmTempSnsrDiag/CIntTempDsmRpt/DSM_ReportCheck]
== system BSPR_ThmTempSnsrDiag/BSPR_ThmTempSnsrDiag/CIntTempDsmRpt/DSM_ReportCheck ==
  note: Fault report to diagnostic management system
  Dfc_id_nv : Inport  OutDataTypeStr=uint8
  Err : Inport  Port=2
  Heal : Inport  Port=3
  Bit Clear1 : simulink/Logic and Bit Operations/Bit Clear  iBit=4
  Bit Clear2 : simulink/Logic and Bit Operations/Bit Clear  iBit=3
  Bit Set : simulink/Logic and Bit Operations/Bit Set  iBit=4
  Bit Set1 : simulink/Logic and Bit Operations/Bit Set  iBit=3
  Bit Set2 : simulink/Logic and Bit Operations/Bit Set  iBit=3
  Bit Set4 : simulink/Logic and Bit Operations/Bit Set  iBit=7
  Constant7 : Constant  Value=0  OutDataTypeStr=boolean
  Delay2 : Delay  DelayLength=1  InitialCondition=1
  Delay3 : Delay  DelayLength=1  InitialCondition=0
  Switch2 : Switch  Criteria=u2 ~= 0
  Switch3 : Switch  Criteria=u2 ~= 0
  Switch4 : Switch  Criteria=u2 ~= 0
  Dfc_id : Outport  OutDataTypeStr=uint8
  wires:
  Dfc_id_nv/1 -> Bit Clear2/1, Bit Set4/1, Bit Clear1/1
  Bit Set4/1 -> Bit Set/1
  Constant7/1 -> Delay2/1
  Delay2/1 -> Switch2/2
  Switch3/1 -> Switch2/3
  Bit Clear2/1 -> Switch2/1
  Switch2/1 -> Delay3/1, Dfc_id/1
  Bit Set1/1 -> Switch3/1
  Bit Set/1 -> Bit Set1/1
  Switch4/1 -> Switch3/3
  Err/1 -> Switch3/2
  Bit Set2/1 -> Switch4/1
  Bit Clear1/1 -> Bit Set2/1
  Delay3/1 -> Switch4/3
  Heal/1 -> Switch4/2

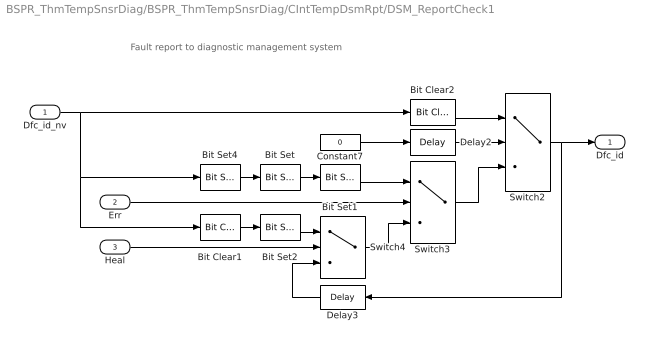
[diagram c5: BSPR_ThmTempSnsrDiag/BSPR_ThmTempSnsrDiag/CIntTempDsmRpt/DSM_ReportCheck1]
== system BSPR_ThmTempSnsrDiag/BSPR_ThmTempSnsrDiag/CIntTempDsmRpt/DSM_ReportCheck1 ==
  note: Fault report to diagnostic management system
  Dfc_id_nv : Inport  OutDataTypeStr=uint8
  Err : Inport  Port=2
  Heal : Inport  Port=3
  Bit Clear1 : simulink/Logic and Bit Operations/Bit Clear  iBit=4
  Bit Clear2 : simulink/Logic and Bit Operations/Bit Clear  iBit=3
  Bit Set : simulink/Logic and Bit Operations/Bit Set  iBit=4
  Bit Set1 : simulink/Logic and Bit Operations/Bit Set  iBit=3
  Bit Set2 : simulink/Logic and Bit Operations/Bit Set  iBit=3
  Bit Set4 : simulink/Logic and Bit Operations/Bit Set  iBit=7
  Constant7 : Constant  Value=0  OutDataTypeStr=boolean
  Delay2 : Delay  DelayLength=1  InitialCondition=1
  Delay3 : Delay  DelayLength=1  InitialCondition=0
  Switch2 : Switch  Criteria=u2 ~= 0
  Switch3 : Switch  Criteria=u2 ~= 0
  Switch4 : Switch  Criteria=u2 ~= 0
  Dfc_id : Outport  OutDataTypeStr=uint8
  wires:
  Heal/1 -> Switch4/2
  Delay3/1 -> Switch4/3
  Bit Clear1/1 -> Bit Set2/1
  Bit Set2/1 -> Switch4/1
  Err/1 -> Switch3/2
  Switch4/1 -> Switch3/3
  Bit Set/1 -> Bit Set1/1
  Bit Set1/1 -> Switch3/1
  Switch2/1 -> Dfc_id/1, Delay3/1
  Bit Clear2/1 -> Switch2/1
  Switch3/1 -> Switch2/3
  Delay2/1 -> Switch2/2
  Constant7/1 -> Delay2/1
  Bit Set4/1 -> Bit Set/1
  Dfc_id_nv/1 -> Bit Clear1/1, Bit Set4/1, Bit Clear2/1

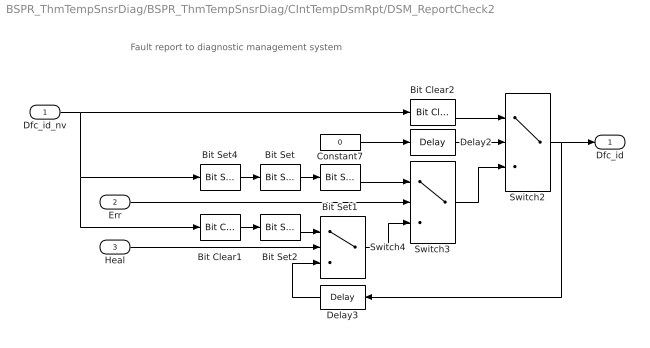
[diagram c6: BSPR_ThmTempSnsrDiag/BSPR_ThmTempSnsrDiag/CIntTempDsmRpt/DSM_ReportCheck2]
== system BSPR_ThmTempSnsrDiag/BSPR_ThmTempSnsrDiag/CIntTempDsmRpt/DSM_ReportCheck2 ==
  note: Fault report to diagnostic management system
  Dfc_id_nv : Inport  OutDataTypeStr=uint8
  Err : Inport  Port=2
  Heal : Inport  Port=3
  Bit Clear1 : simulink/Logic and Bit Operations/Bit Clear  iBit=4
  Bit Clear2 : simulink/Logic and Bit Operations/Bit Clear  iBit=3
  Bit Set : simulink/Logic and Bit Operations/Bit Set  iBit=4
  Bit Set1 : simulink/Logic and Bit Operations/Bit Set  iBit=3
  Bit Set2 : simulink/Logic and Bit Operations/Bit Set  iBit=3
  Bit Set4 : simulink/Logic and Bit Operations/Bit Set  iBit=7
  Constant7 : Constant  Value=0  OutDataTypeStr=boolean
  Delay2 : Delay  DelayLength=1  InitialCondition=1
  Delay3 : Delay  DelayLength=1  InitialCondition=0
  Switch2 : Switch  Criteria=u2 ~= 0
  Switch3 : Switch  Criteria=u2 ~= 0
  Switch4 : Switch  Criteria=u2 ~= 0
  Dfc_id : Outport  OutDataTypeStr=uint8
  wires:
  Dfc_id_nv/1 -> Bit Clear2/1, Bit Set4/1, Bit Clear1/1
  Bit Set4/1 -> Bit Set/1
  Constant7/1 -> Delay2/1
  Delay2/1 -> Switch2/2
  Switch3/1 -> Switch2/3
  Bit Clear2/1 -> Switch2/1
  Switch2/1 -> Delay3/1, Dfc_id/1
  Bit Set1/1 -> Switch3/1
  Bit Set/1 -> Bit Set1/1
  Switch4/1 -> Switch3/3
  Err/1 -> Switch3/2
  Bit Set2/1 -> Switch4/1
  Bit Clear1/1 -> Bit Set2/1
  Delay3/1 -> Switch4/3
  Heal/1 -> Switch4/2

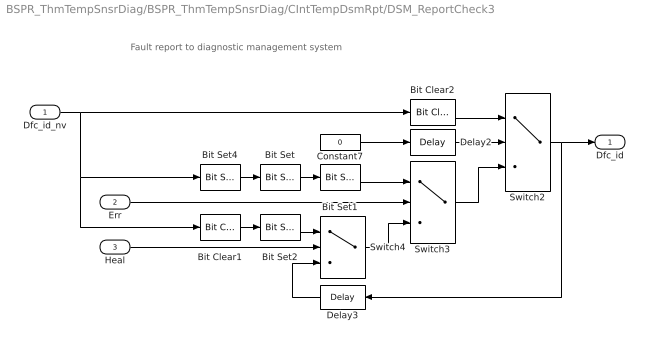
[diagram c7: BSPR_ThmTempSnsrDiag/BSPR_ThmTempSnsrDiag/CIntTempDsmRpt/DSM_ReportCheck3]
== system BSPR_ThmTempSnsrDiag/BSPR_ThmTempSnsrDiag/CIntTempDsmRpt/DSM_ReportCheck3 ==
  note: Fault report to diagnostic management system
  Dfc_id_nv : Inport  OutDataTypeStr=uint8
  Err : Inport  Port=2
  Heal : Inport  Port=3
  Bit Clear1 : simulink/Logic and Bit Operations/Bit Clear  iBit=4
  Bit Clear2 : simulink/Logic and Bit Operations/Bit Clear  iBit=3
  Bit Set : simulink/Logic and Bit Operations/Bit Set  iBit=4
  Bit Set1 : simulink/Logic and Bit Operations/Bit Set  iBit=3
  Bit Set2 : simulink/Logic and Bit Operations/Bit Set  iBit=3
  Bit Set4 : simulink/Logic and Bit Operations/Bit Set  iBit=7
  Constant7 : Constant  Value=0  OutDataTypeStr=boolean
  Delay2 : Delay  DelayLength=1  InitialCondition=1
  Delay3 : Delay  DelayLength=1  InitialCondition=0
  Switch2 : Switch  Criteria=u2 ~= 0
  Switch3 : Switch  Criteria=u2 ~= 0
  Switch4 : Switch  Criteria=u2 ~= 0
  Dfc_id : Outport  OutDataTypeStr=uint8
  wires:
  Heal/1 -> Switch4/2
  Delay3/1 -> Switch4/3
  Bit Clear1/1 -> Bit Set2/1
  Bit Set2/1 -> Switch4/1
  Err/1 -> Switch3/2
  Switch4/1 -> Switch3/3
  Bit Set/1 -> Bit Set1/1
  Bit Set1/1 -> Switch3/1
  Switch2/1 -> Dfc_id/1, Delay3/1
  Bit Clear2/1 -> Switch2/1
  Switch3/1 -> Switch2/3
  Delay2/1 -> Switch2/2
  Constant7/1 -> Delay2/1
  Bit Set4/1 -> Bit Set/1
  Dfc_id_nv/1 -> Bit Clear1/1, Bit Set4/1, Bit Clear2/1

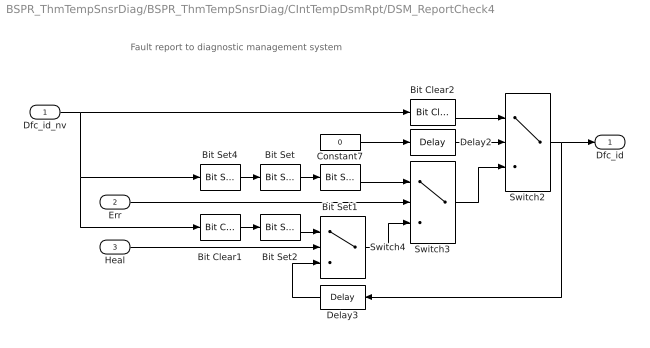
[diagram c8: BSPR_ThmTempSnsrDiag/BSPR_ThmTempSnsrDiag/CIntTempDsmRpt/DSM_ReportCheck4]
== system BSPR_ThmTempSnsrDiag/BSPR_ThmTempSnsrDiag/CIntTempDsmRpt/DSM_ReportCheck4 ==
  note: Fault report to diagnostic management system
  Dfc_id_nv : Inport  OutDataTypeStr=uint8
  Err : Inport  Port=2
  Heal : Inport  Port=3
  Bit Clear1 : simulink/Logic and Bit Operations/Bit Clear  iBit=4
  Bit Clear2 : simulink/Logic and Bit Operations/Bit Clear  iBit=3
  Bit Set : simulink/Logic and Bit Operations/Bit Set  iBit=4
  Bit Set1 : simulink/Logic and Bit Operations/Bit Set  iBit=3
  Bit Set2 : simulink/Logic and Bit Operations/Bit Set  iBit=3
  Bit Set4 : simulink/Logic and Bit Operations/Bit Set  iBit=7
  Constant7 : Constant  Value=0  OutDataTypeStr=boolean
  Delay2 : Delay  DelayLength=1  InitialCondition=1
  Delay3 : Delay  DelayLength=1  InitialCondition=0
  Switch2 : Switch  Criteria=u2 ~= 0
  Switch3 : Switch  Criteria=u2 ~= 0
  Switch4 : Switch  Criteria=u2 ~= 0
  Dfc_id : Outport  OutDataTypeStr=uint8
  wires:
  Dfc_id_nv/1 -> Bit Clear2/1, Bit Set4/1, Bit Clear1/1
  Bit Set4/1 -> Bit Set/1
  Constant7/1 -> Delay2/1
  Delay2/1 -> Switch2/2
  Switch3/1 -> Switch2/3
  Bit Clear2/1 -> Switch2/1
  Switch2/1 -> Delay3/1, Dfc_id/1
  Bit Set1/1 -> Switch3/1
  Bit Set/1 -> Bit Set1/1
  Switch4/1 -> Switch3/3
  Err/1 -> Switch3/2
  Bit Set2/1 -> Switch4/1
  Bit Clear1/1 -> Bit Set2/1
  Delay3/1 -> Switch4/3
  Heal/1 -> Switch4/2

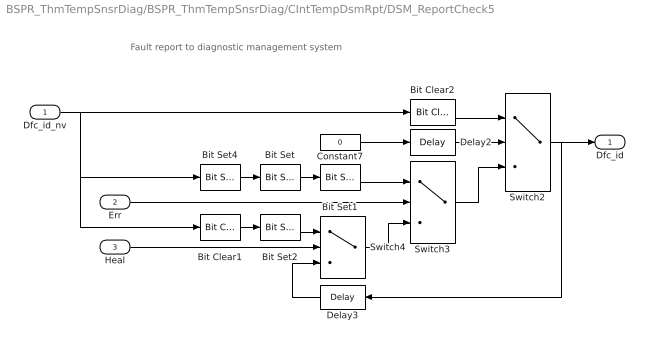
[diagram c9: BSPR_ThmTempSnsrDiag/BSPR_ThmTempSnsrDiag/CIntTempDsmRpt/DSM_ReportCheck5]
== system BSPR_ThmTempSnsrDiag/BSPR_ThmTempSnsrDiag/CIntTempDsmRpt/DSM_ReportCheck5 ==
  note: Fault report to diagnostic management system
  Dfc_id_nv : Inport  OutDataTypeStr=uint8
  Err : Inport  Port=2
  Heal : Inport  Port=3
  Bit Clear1 : simulink/Logic and Bit Operations/Bit Clear  iBit=4
  Bit Clear2 : simulink/Logic and Bit Operations/Bit Clear  iBit=3
  Bit Set : simulink/Logic and Bit Operations/Bit Set  iBit=4
  Bit Set1 : simulink/Logic and Bit Operations/Bit Set  iBit=3
  Bit Set2 : simulink/Logic and Bit Operations/Bit Set  iBit=3
  Bit Set4 : simulink/Logic and Bit Operations/Bit Set  iBit=7
  Constant7 : Constant  Value=0  OutDataTypeStr=boolean
  Delay2 : Delay  DelayLength=1  InitialCondition=1
  Delay3 : Delay  DelayLength=1  InitialCondition=0
  Switch2 : Switch  Criteria=u2 ~= 0
  Switch3 : Switch  Criteria=u2 ~= 0
  Switch4 : Switch  Criteria=u2 ~= 0
  Dfc_id : Outport  OutDataTypeStr=uint8
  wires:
  Heal/1 -> Switch4/2
  Delay3/1 -> Switch4/3
  Bit Clear1/1 -> Bit Set2/1
  Bit Set2/1 -> Switch4/1
  Err/1 -> Switch3/2
  Switch4/1 -> Switch3/3
  Bit Set/1 -> Bit Set1/1
  Bit Set1/1 -> Switch3/1
  Switch2/1 -> Dfc_id/1, Delay3/1
  Bit Clear2/1 -> Switch2/1
  Switch3/1 -> Switch2/3
  Delay2/1 -> Switch2/2
  Constant7/1 -> Delay2/1
  Bit Set4/1 -> Bit Set/1
  Dfc_id_nv/1 -> Bit Clear1/1, Bit Set4/1, Bit Clear2/1

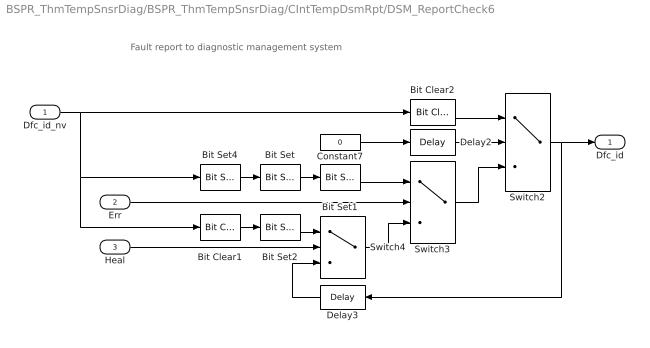
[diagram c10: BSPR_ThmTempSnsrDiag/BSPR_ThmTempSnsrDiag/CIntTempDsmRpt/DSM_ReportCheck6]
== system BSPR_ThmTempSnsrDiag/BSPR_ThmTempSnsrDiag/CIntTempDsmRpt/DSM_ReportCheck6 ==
  note: Fault report to diagnostic management system
  Dfc_id_nv : Inport  OutDataTypeStr=uint8
  Err : Inport  Port=2
  Heal : Inport  Port=3
  Bit Clear1 : simulink/Logic and Bit Operations/Bit Clear  iBit=4
  Bit Clear2 : simulink/Logic and Bit Operations/Bit Clear  iBit=3
  Bit Set : simulink/Logic and Bit Operations/Bit Set  iBit=4
  Bit Set1 : simulink/Logic and Bit Operations/Bit Set  iBit=3
  Bit Set2 : simulink/Logic and Bit Operations/Bit Set  iBit=3
  Bit Set4 : simulink/Logic and Bit Operations/Bit Set  iBit=7
  Constant7 : Constant  Value=0  OutDataTypeStr=boolean
  Delay2 : Delay  DelayLength=1  InitialCondition=1
  Delay3 : Delay  DelayLength=1  InitialCondition=0
  Switch2 : Switch  Criteria=u2 ~= 0
  Switch3 : Switch  Criteria=u2 ~= 0
  Switch4 : Switch  Criteria=u2 ~= 0
  Dfc_id : Outport  OutDataTypeStr=uint8
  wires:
  Dfc_id_nv/1 -> Bit Clear2/1, Bit Set4/1, Bit Clear1/1
  Bit Set4/1 -> Bit Set/1
  Constant7/1 -> Delay2/1
  Delay2/1 -> Switch2/2
  Switch3/1 -> Switch2/3
  Bit Clear2/1 -> Switch2/1
  Switch2/1 -> Delay3/1, Dfc_id/1
  Bit Set1/1 -> Switch3/1
  Bit Set/1 -> Bit Set1/1
  Switch4/1 -> Switch3/3
  Err/1 -> Switch3/2
  Bit Set2/1 -> Switch4/1
  Bit Clear1/1 -> Bit Set2/1
  Delay3/1 -> Switch4/3
  Heal/1 -> Switch4/2

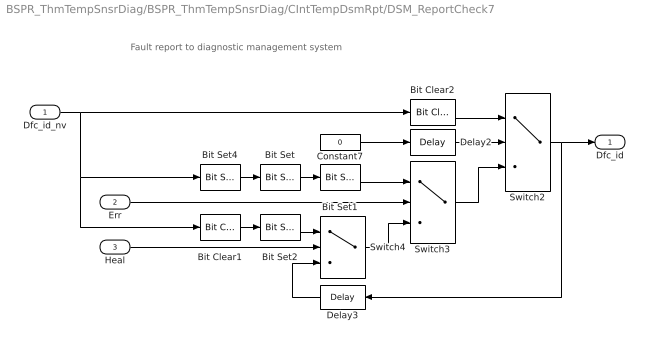
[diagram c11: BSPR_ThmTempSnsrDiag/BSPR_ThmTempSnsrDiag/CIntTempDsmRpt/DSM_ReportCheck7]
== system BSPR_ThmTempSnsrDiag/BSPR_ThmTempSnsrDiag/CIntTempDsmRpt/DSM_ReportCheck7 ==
  note: Fault report to diagnostic management system
  Dfc_id_nv : Inport  OutDataTypeStr=uint8
  Err : Inport  Port=2
  Heal : Inport  Port=3
  Bit Clear1 : simulink/Logic and Bit Operations/Bit Clear  iBit=4
  Bit Clear2 : simulink/Logic and Bit Operations/Bit Clear  iBit=3
  Bit Set : simulink/Logic and Bit Operations/Bit Set  iBit=4
  Bit Set1 : simulink/Logic and Bit Operations/Bit Set  iBit=3
  Bit Set2 : simulink/Logic and Bit Operations/Bit Set  iBit=3
  Bit Set4 : simulink/Logic and Bit Operations/Bit Set  iBit=7
  Constant7 : Constant  Value=0  OutDataTypeStr=boolean
  Delay2 : Delay  DelayLength=1  InitialCondition=1
  Delay3 : Delay  DelayLength=1  InitialCondition=0
  Switch2 : Switch  Criteria=u2 ~= 0
  Switch3 : Switch  Criteria=u2 ~= 0
  Switch4 : Switch  Criteria=u2 ~= 0
  Dfc_id : Outport  OutDataTypeStr=uint8
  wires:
  Heal/1 -> Switch4/2
  Delay3/1 -> Switch4/3
  Bit Clear1/1 -> Bit Set2/1
  Bit Set2/1 -> Switch4/1
  Err/1 -> Switch3/2
  Switch4/1 -> Switch3/3
  Bit Set/1 -> Bit Set1/1
  Bit Set1/1 -> Switch3/1
  Switch2/1 -> Dfc_id/1, Delay3/1
  Bit Clear2/1 -> Switch2/1
  Switch3/1 -> Switch2/3
  Delay2/1 -> Switch2/2
  Constant7/1 -> Delay2/1
  Bit Set4/1 -> Bit Set/1
  Dfc_id_nv/1 -> Bit Clear1/1, Bit Set4/1, Bit Clear2/1

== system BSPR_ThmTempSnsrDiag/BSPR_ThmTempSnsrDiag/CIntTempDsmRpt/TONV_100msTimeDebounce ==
  note: Turn On Delay Time Deboune
  u : Inport
  T : Inport  Port=2
  Add : Sum
  Constant1 : Constant  Value=0  OutDataTypeStr=single
  Constant2 : Constant  OutDataTypeStr=uint8
  Constant3 : Constant  Value=0  OutDataTypeStr=uint8
  Constant4 : Constant  Value=0.1  OutDataTypeStr=single
  Delay : Delay  DelayLength=1  InitialCondition=0
  MinMax : MinMax  Inputs=2
  Product : Product  OutMin=[0]  OutMax=[65535]  OutDataTypeStr=single
  Relational Operator : RelationalOperator  Operator=>  OutDataTypeStr=boolean  RndMeth=Simplest
  Switch : Switch  Criteria=u2 ~= 0
  Switch1 : Switch  Criteria=u2 ~= 0
  y : Outport
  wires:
  Switch1/1 -> Product/1
  Constant3/1 -> Switch1/3
  Constant2/1 -> Switch1/1
  u/1 -> Switch1/2, Switch/2
  Constant4/1 -> Switch/1
  Constant1/1 -> Switch/3
  Add/1 -> Product/2
  Product/1 -> Relational Operator/1, Delay/1
  Switch/1 -> Add/1
  Delay/1 -> MinMax/2
  Relational Operator/1 -> y/1
  T/1 -> MinMax/1, Relational Operator/2
  MinMax/1 -> Add/2

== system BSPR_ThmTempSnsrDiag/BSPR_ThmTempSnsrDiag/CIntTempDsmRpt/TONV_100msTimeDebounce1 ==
  note: Turn On Delay Time Deboune
  u : Inport
  T : Inport  Port=2
  Add : Sum
  Constant1 : Constant  Value=0  OutDataTypeStr=single
  Constant2 : Constant  OutDataTypeStr=uint8
  Constant3 : Constant  Value=0  OutDataTypeStr=uint8
  Constant4 : Constant  Value=0.1  OutDataTypeStr=single
  Delay : Delay  DelayLength=1  InitialCondition=0
  MinMax : MinMax  Inputs=2
  Product : Product  OutMin=[0]  OutMax=[65535]  OutDataTypeStr=single
  Relational Operator : RelationalOperator  Operator=>  OutDataTypeStr=boolean  RndMeth=Simplest
  Switch : Switch  Criteria=u2 ~= 0
  Switch1 : Switch  Criteria=u2 ~= 0
  y : Outport
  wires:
  MinMax/1 -> Add/2
  T/1 -> Relational Operator/2, MinMax/1
  Relational Operator/1 -> y/1
  Delay/1 -> MinMax/2
  Switch/1 -> Add/1
  Product/1 -> Delay/1, Relational Operator/1
  Add/1 -> Product/2
  Constant1/1 -> Switch/3
  Constant4/1 -> Switch/1
  u/1 -> Switch/2, Switch1/2
  Constant2/1 -> Switch1/1
  Constant3/1 -> Switch1/3
  Switch1/1 -> Product/1

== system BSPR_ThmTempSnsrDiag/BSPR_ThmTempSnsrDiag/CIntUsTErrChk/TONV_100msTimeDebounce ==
  note: Turn On Delay Time Deboune
  u : Inport
  T : Inport  Port=2
  Add : Sum
  Constant1 : Constant  Value=0  OutDataTypeStr=single
  Constant2 : Constant  OutDataTypeStr=uint8
  Constant3 : Constant  Value=0  OutDataTypeStr=uint8
  Constant4 : Constant  Value=0.1  OutDataTypeStr=single
  Delay : Delay  DelayLength=1  InitialCondition=0
  MinMax : MinMax  Inputs=2
  Product : Product  OutMin=[0]  OutMax=[65535]  OutDataTypeStr=single
  Relational Operator : RelationalOperator  Operator=>  OutDataTypeStr=boolean  RndMeth=Simplest
  Switch : Switch  Criteria=u2 ~= 0
  Switch1 : Switch  Criteria=u2 ~= 0
  y : Outport
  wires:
  Switch1/1 -> Product/1
  Constant3/1 -> Switch1/3
  Constant2/1 -> Switch1/1
  u/1 -> Switch1/2, Switch/2
  Constant4/1 -> Switch/1
  Constant1/1 -> Switch/3
  Add/1 -> Product/2
  Product/1 -> Relational Operator/1, Delay/1
  Switch/1 -> Add/1
  Delay/1 -> MinMax/2
  Relational Operator/1 -> y/1
  T/1 -> MinMax/1, Relational Operator/2
  MinMax/1 -> Add/2
